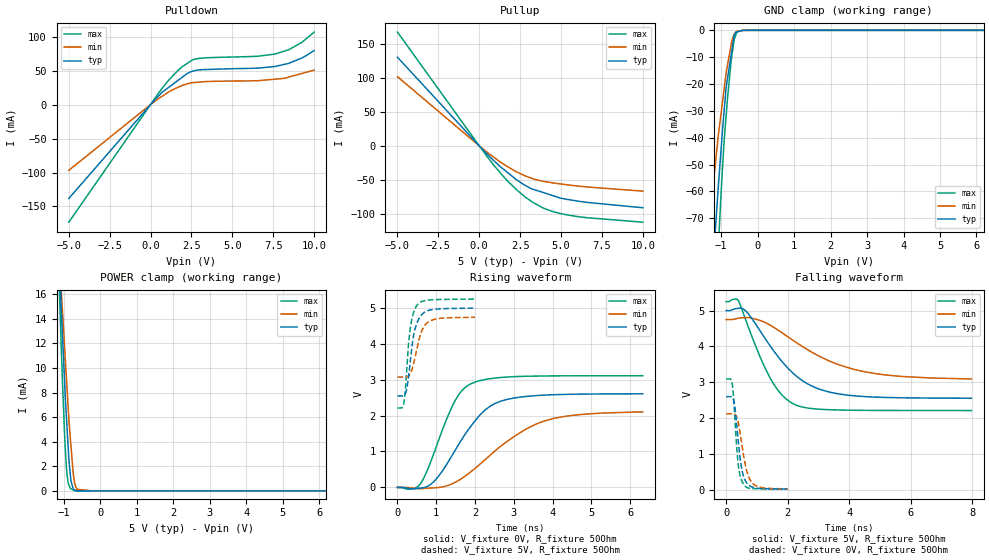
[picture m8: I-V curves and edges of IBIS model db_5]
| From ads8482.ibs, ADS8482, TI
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|   db_5 Model
[Model]   db_5
Model_type   3-state
Polarity   Non-Inverting
Vmeas = 2.5
Vref = 2.5
Cref = 5pF
Rref = 50
|   typ   min   max
|   (nom PVT)   (Fast PVT)   (slow PVT)
|C_comp from frequency method(F=1MHz)
|Average
|C_comp   3.586e-11   1.876e-11   6.842e-11
|ON state : BUFFER OUTPUT TURNED HIGH
|C_comp   3.586e-11   1.876e-11   6.842e-11
|OFF state: BUFFER IN HIGH IMPEDANCE
|C_comp   2.904e-12   2.164e-12   3.664e-12
|C_comp from L-C Tank method(L=1nH)
|Resonant Frequency(Hz)   3.49e9   3.93e9   3.16e9
C_comp   2.082e-12   1.642e-12   2.539e-12
| Where nom  PVT is Nominal Process,  5V,  30C
|   Fast PVT is Strong Process,   5.25V,  -40C
|   Slow PVT is Weak Process,   4.75V,  90C
[Voltage Range]   5   4.75   5.25
|Ambient Temperature   25   85   -40
|Junction Temperature
[Temperature Range]   30   90   -40
[Pullup Reference]   5   4.75   5.25
[Pulldown Reference]   0   0   0
[Power Clamp Reference]   5   4.75   5.25
[GND Clamp Reference]   0   0   0
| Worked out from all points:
|   slope of the pulldown table from 0 to 0.75 V, typ, clamps not added: 39.6 ohm
|   slope of the pullup table from 0 to 0.75 V, typ, clamps not added: 40.4 ohm
|   GND clamp passes 1 mA (typ) near -0.61 V on its own axis
|   POWER clamp passes 1 mA (typ) near -0.81 V on its own axis
|   falling waveform, V_fixture 5V, R_fixture 50Ohm: 20-80 % time 1.43ns typ, 2.14ns min, 970ps max; typ from 5 V to 2.55 V
|   rising waveform, V_fixture 0V, R_fixture 50Ohm: 20-80 % time 995ps typ, 1.55ns min, 701ps max; typ from 0 V to 2.61 V
|   rising waveform, V_fixture 5V, R_fixture 50Ohm: 20-80 % time 198ps typ, 239ps min, 153ps max; typ from 2.55 V to 4.99 V
|   falling waveform, V_fixture 0V, R_fixture 50Ohm: 20-80 % time 204ps typ, 265ps min, 156ps max; typ from 2.6 V to 0.014 V
[Pulldown]
|   Voltage   I(typ)   I(min)   I(max)
-5V       -138.2mA   -96.8mA    -173.1mA
255mV     6.939mA    4.817mA    8.895mA
1.097V    25.2mA     18.42mA    35.57mA
1.921V    40.01mA    27.94mA    55.46mA
2.27V     46.27mA    30.77mA    61.1mA
2.572V    49.12mA    32.25mA    66mA
2.94V     50.91mA    33mA       68mA
6.557V    53.68mA    35.17mA    71.19mA
7.591V    55.97mA    37.39mA    74.28mA
8.442V    60.69mA    40.48mA    80.67mA
9.229V    68.39mA    45.68mA    91.25mA
10V       79.5mA     50.78mA    106.7mA
[GND Clamp]
|   Voltage   I(typ)   I(min)   I(max)
-5V       -964.4mA   -707.2mA   -1.308A
-1.51V    -147.6mA   -97.97mA   -211.3mA
-1.31V    -104.8mA   -69.35mA   -149.7mA
-1.165V   -75.75mA   -50.59mA   -106.4mA
-1.055V   -54.09mA   -36.7mA    -74.85mA
-924mV    -30.92mA   -22.45mA   -42.42mA
-865mV    -21.33mA   -16.04mA   -32.09mA
-824.3mV  -17.77mA   -12.84mA   -25.15mA
-714mV    -8.153mA   -4.435mA   -9.969mA
-640mV    -1.696mA   -1.423mA   -3.33mA
-579.5mV  -607.3uA   -377.8uA   -1.011mA
10V       0A         0A         0A
[Pullup]
|   Voltage   I(typ)   I(min)   I(max)
-5V       130.2mA    101.7mA    167.2mA
561.7mV   -14.1mA    -10.88mA   -18.36mA
1.235V    -29.57mA   -22.86mA   -38.21mA
1.596V    -36.57mA   -28.63mA   -48.1mA
2.27V     -49.64mA   -38.06mA   -64.07mA
2.793V    -57.82mA   -44.04mA   -74.8mA
3.165V    -62.81mA   -47.26mA   -81.17mA
3.838V    -68.04mA   -51.69mA   -90.54mA
4.956V    -76.73mA   -55.96mA   -99.47mA
6.56V     -83.02mA   -60.34mA   -105.6mA
10V       -90.89mA   -66.6mA    -112.2mA
[POWER Clamp]
|   Voltage   I(typ)   I(min)   I(max)
-5V       186.5mA    166.7mA    213.4mA
-1.306V   31.73mA    29.63mA    33.26mA
-1.103V   17.02mA    18.02mA    14.49mA
-1.085V   15.76mA    17.06mA    12.99mA
-1.04V    12.81mA    14.74mA    9.128mA
-981.8mV  9.094mA    11.85mA    4.789mA
-913.5mV  5.223mA    8.438mA    1.356mA
-860mV    2.55mA     5.76mA     477.6uA
-805mV    829.9uA    3.691mA    177.7uA
-698.3mV  76.98uA    558.1uA    8.233uA
-190mV    0A         0A         431.6nA
10V       0A         0A         0A
[Ramp]
R_load = 50
|   typ   min   max
dV/dt_r   1.56464/9.93778e-10   1.27123/1.56137e-09   1.86541/7.01462e-10
dV/dt_f   1.46902/1.43454e-09   0.995787/2.14411e-09   1.82539/9.70001e-10
[Falling Waveform]
V_fixture = 5V
V_fixture_min = 4.75V
V_fixture_max = 5.25V
R_fixture = 50Ohm
|   Time   V(typ)   V(min)   V(max)
0s        5V         4.75V      5.25V
400ps     5.064V     4.788V     5.279V
700ps     4.932V     4.807V     4.594V
1.075ns   4.474V     4.735V     3.767V
1.425ns   4.022V     4.597V     3.129V
1.825ns   3.568V     4.376V     2.634V
2.25ns    3.194V     4.126V     2.369V
3.1ns     2.785V     3.694V     2.241V
4.475ns   2.599V     3.298V     2.213V
7.975ns   2.552V     3.09V      2.208V
[Rising Waveform]
V_fixture = 0V
V_fixture_min = 0V
V_fixture_max = 0V
R_fixture = 50Ohm
|   Time   V(typ)   V(min)   V(max)
0s        1.773nV    2.079nV    1.568nV
425ps     -40.28mV   -22.59mV   -25.26mV
600ps     -18.98mV   -34.77mV   115.1mV
950ps     176.5mV    -11.21mV   984.1mV
1.45ns    965.1mV    121.2mV    2.34V
1.875ns   1.678V     420.6mV    2.874V
2.525ns   2.34V      1.024V     3.045V
3.75ns    2.566V     1.836V     3.101V
4.55ns    2.593V     2.009V     3.106V
6.325ns   2.606V     2.103V     3.109V
[Rising Waveform]
V_fixture = 5V
V_fixture_min = 4.75V
V_fixture_max = 5.25V
R_fixture = 50Ohm
|   Time   V(typ)   V(min)   V(max)
0s        2.548V     3.071V     2.207V
162ps     2.555V     3.071V     2.322V
194ps     2.588V     3.071V     2.603V
242ps     2.758V     3.074V     3.305V
324ps     3.437V     3.151V     4.373V
406ps     4.166V     3.4V       4.833V
495ps     4.555V     3.826V     5.057V
639ps     4.823V     4.388V     5.177V
839ps     4.937V     4.631V     5.217V
1.999ns   4.987V     4.735V     5.241V
[Falling Waveform]
V_fixture = 0V
V_fixture_min = 0V
V_fixture_max = 0V
R_fixture = 50Ohm
|   Time   V(typ)   V(min)   V(max)
0s        2.595V     2.117V     3.089V
142ps     2.596V     2.117V     3.091V
198ps     2.581V     2.118V     2.952V
278ps     2.343V     2.104V     2.083V
382ps     1.477V     1.915V     796.9mV
447ps     931.8mV    1.621V     414.1mV
532ps     477.4mV    1.145V     198.3mV
686ps     167mV      466.4mV    52.71mV
872ps     59.45mV    163.2mV    26.2mV
1.999ns   14.1mV     17.42mV    9.905mV
